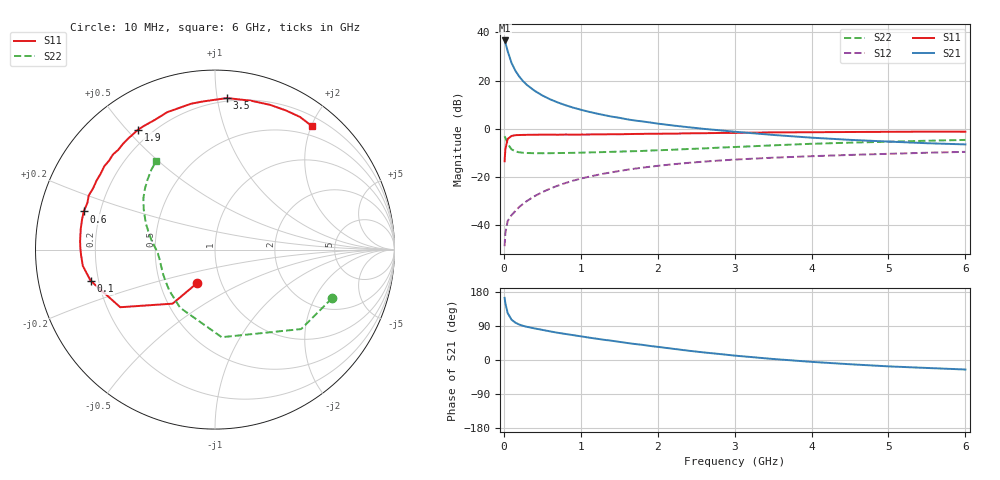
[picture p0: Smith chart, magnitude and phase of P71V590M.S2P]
! SIEMENS Small Signal Semiconductors
! BFP196
! Si NPN RF Bipolar Junction Transistor in SOT143
! VCE = 1.5 V  IC = 90 mA
! Common Emitter S-Parameters:  May  1996
# GHz  S  MA  R  50
!  f  S11  S21  S12  S22
! GHz  MAG  ANG  MAG  ANG  MAG  ANG  MAG  ANG
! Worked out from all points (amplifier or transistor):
!   36 points, 10 MHz to 6 GHz, reference 50 ohm
!   highest |S21| = 36.7 dB at 10 MHz (marker M1)
!   |S21| within 3 dB of that: start of sweep to 37.5 MHz
!   unconditionally stable (mu >= 1): 249 MHz to end of sweep
!   at 250 MHz: K = 1.00, MAG = 25.2 dB, |S12| = -31.1 dB
!   at 1.4 GHz: K = 1.12, MAG = 9.4 dB, |S12| = -18.0 dB
!   at 6 GHz: K = 1.03, MAG = 0.5 dB, |S12| = -9.5 dB
!   S11 on the Smith chart (normalised r, x): 10 MHz: 0.76, -0.30; 100 MHz: 0.17, -0.12; 600 MHz: 0.14, +0.14; 1.9 GHz: 0.15, +0.54; 3.5 GHz: 0.18, +1.07; 6 GHz: 0.34, +2.01
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0.01  0.2139 -118.4  68.29 164.0  0.0037 70.9  0.7057 -22.6
0.02  0.3826 -128.1  61.39 149.4  0.007 62.4  0.6529 -42.7
0.05  0.6181 -148.7  40.76 123.8  0.0123 50.6  0.4895 -85.6
0.1  0.7141 -165.9  23.36 106.4  0.0163 50.2  0.3778 -121.0
0.15  0.7421 -173.0  16.08 98.5  0.0198 54.6  0.3419 -138.0
0.2  0.7467 -177.6  12.2 93.6  0.0241 58.6  0.3269 -147.6
0.25  0.751 178.8  9.757 90.2  0.0278 61.2  0.3201 -154.3
0.3  0.7532 176.3  8.172 87.6  0.032 62.9  0.3166 -158.4
0.4  0.7567 171.4  6.177 83.3  0.0404 65.8  0.3134 -164.4
0.5  0.7595 167.5  4.943 79.5  0.0487 66.7  0.313 -168.1
0.6  0.7617 163.8  4.119 75.6  0.0577 66.5  0.3138 -170.8
0.7  0.7571 159.9  3.544 71.8  0.0665 66.1  0.3157 -172.9
0.8  0.7654 156.8  3.107 68.8  0.0753 65.0  0.3173 -174.5
1.1  0.7649 146.3  2.279 59.3  0.1015 62.0  0.3252 -178.7
1.4  0.7773 137.0  1.801 50.9  0.1259 57.5  0.3343 177.9
1.9  0.7938 122.7  1.361 37.1  0.1643 49.7  0.3554 172.2
2.2  0.7971 114.7  1.176 29.6  0.1849 44.8  0.3701 168.3
2.8  0.8234 99.4  0.938 15.9  0.2207 35.5  0.4089 159.9
3.5  0.8468 85.5  0.75 2.7  0.2531 25.1  0.4563 150.5
4.5  0.8628 69.2  0.593 -11.2  0.2887 12.8  0.5186 138.7
5.5  0.8778 57.3  0.505 -21.0  0.3204 2.0  0.5684 128.7
6  0.8745 51.9  0.477 -25.1  0.3345 -3.9  0.5912 123.7
